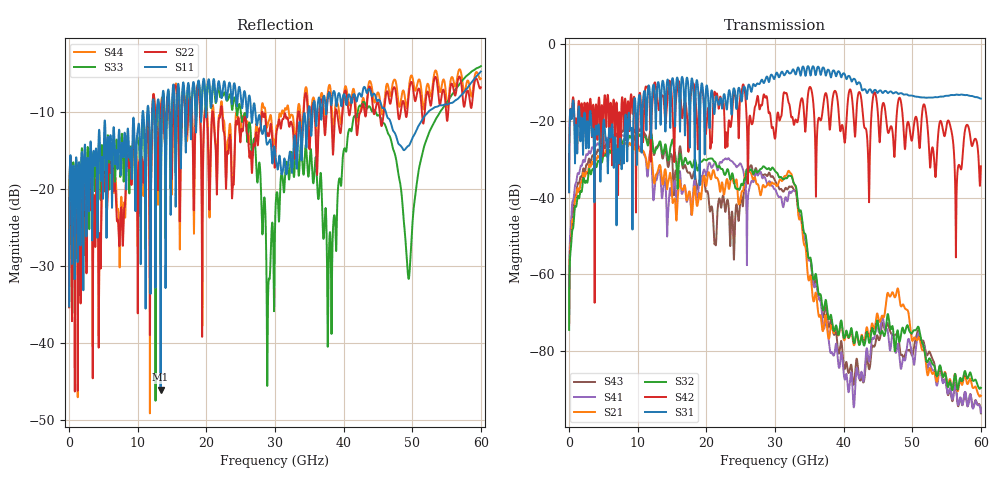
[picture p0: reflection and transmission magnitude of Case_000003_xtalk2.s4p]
! Info: Touchstone file created by circ.  Input file=CasetestDOE_NRZ_template_000003.circ
# Hz S RI R 50
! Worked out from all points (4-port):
!   6000 points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, 10 MHz to 60 GHz, reference 50 ohm
!   strongest paths, dB at 10 MHz, 15.01 GHz, 30.01 GHz, 45.01 GHz, 60 GHz:
!     S31: -38.6, -9.1, -8.5, -12.6, -14.1
!     S42: -38.6, -14.8, -24.6, -18.3, -31.8
!     S32: -74.5, -25.1, -33.0, -72.7, -89.6
!     S21: -73.1, -39.1, -36.3, -70.8, -91.7
!     S41: -70.3, -38.9, -37.8, -74.1, -96.0
!     S43: -72.6, -29.5, -35.5, -76.5, -96.3
!   lowest |S11| = -46.1 dB at 13.34 GHz (marker M1), VSWR 1.01, Z = 50.1 + j0.485 ohm
!   |S11| at or under -10 dB: start of sweep to 10.72 GHz; 27.14 GHz to 34.84 GHz (7.705 GHz wide, 24.9 % of centre); 46.16 GHz to 52.31 GHz (6.155 GHz wide, 12.5 % of centre)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
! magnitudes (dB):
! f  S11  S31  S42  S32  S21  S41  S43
! 10 MHz  -35.2  -38.6  -38.6  -74.5  -73.1  -70.3  -72.6
! 3.56 GHz  -15.2  -23.4  -16.1  -32.6  -31.4  -27.1  -29.0
! 13.34 GHz  -46.1  -21.0  -14.1  -25.6  -32.2  -34.8  -26.5
! 32.84 GHz  -13.2  -7.2  -20.7  -36.5  -36.6  -38.1  -38.1
! 38.23 GHz  -9.1  -8.2  -17.2  -71.1  -73.2  -80.3  -71.9
! 49.47 GHz  -14.4  -13.3  -20.5  -74.2  -70.3  -76.8  -79.8
! 60 GHz  -4.7  -14.1  -31.8  -89.6  -91.7  -96.0  -96.3
